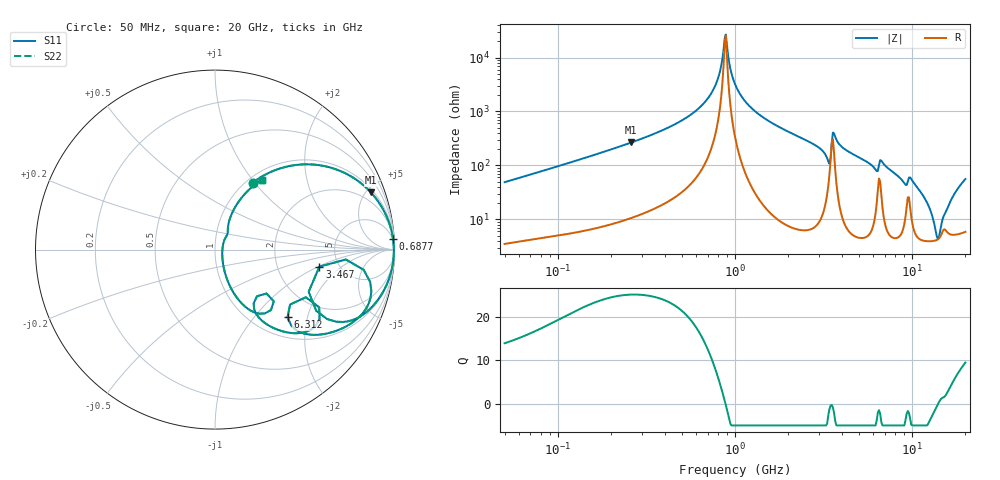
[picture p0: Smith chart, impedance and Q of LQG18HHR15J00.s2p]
!Murata Part Number: LQG18HHR15J00
!These Parameters are Measured in Series Mode Connection
!  o--[Z]--o
!Port1  Port2
!  o-------o
!Freq. Start=50[MHz] Stop=20[GHz], 401[Steps]
# Hz S RI R 50
!Freq.(Hz) S11(Real) S11(Imag) S21(Real) S21(Imag) S12(Real) S12(Imag) S22(Real) S22(Imag)
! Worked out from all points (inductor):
!   401 points, 50 MHz to 20 GHz, reference 50 ohm
!   read as one part in series: L = 153 nH near 51.52 MHz
!   highest Q = 25.1 at 259.7 MHz (marker M1), where L = 163 nH
!   self-resonance near 873.9 MHz
!   S11 on the Smith chart (normalised r, x): 50 MHz: 1.07, +0.98; 687.7 MHz: 3, +32; 3.467 GHz: 3.55, -1.03; 6.312 GHz: 1.40, -1.52; 20 GHz: 1.12, +1.12
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5e7  0.2095 0.3726  0.7905 -0.3726  0.7905 -0.3726  0.2095 0.3726
1.364002e8  0.631 0.4603  0.369 -0.4603  0.369 -0.4603  0.631 0.4603
2.597386e8  0.8669 0.3203  0.1331 -0.3203  0.1331 -0.3203  0.8669 0.3203
3.721004e8  0.9385 0.2206  0.0615 -0.2206  0.0615 -0.2206  0.9385 0.2206
6.87656e8  0.9915 0.0615  0.00849 -0.0615  0.00849 -0.0615  0.9915 0.0615
7.868965e8  0.9952 0.0284  0.00484 -0.0284  0.00484 -0.0284  0.9952 0.0284
8.870719e8  0.9964 -0.000985  0.00359 0.000985  0.00359 0.000985  0.9964 -0.000985
1e9  0.9958 -0.0306  0.00421 0.0306  0.00421 0.0306  0.9958 -0.0306
1.369645e9  0.9843 -0.1118  0.0157 0.1118  0.0157 0.1118  0.9843 -0.1118
2.728004e9  0.861 -0.3331  0.139 0.3331  0.139 0.3331  0.861 -0.3331
3.216634e9  0.7123 -0.4034  0.2877 0.4034  0.2877 0.4034  0.7123 -0.4034
3.466789e9  0.5817 -0.0949  0.4183 0.0949  0.4183 0.0949  0.5817 -0.0949
3.736399e9  0.8662 -0.27  0.1338 0.27  0.1338 0.27  0.8662 -0.27
5.194772e9  0.6327 -0.4654  0.3673 0.4654  0.3673 0.4654  0.6327 -0.4654
6.311513e9  0.404 -0.3774  0.596 0.3774  0.596 0.3774  0.404 -0.3774
6.802353e9  0.5577 -0.4282  0.4423 0.4282  0.4423 0.4282  0.5577 -0.4282
7.442007e9  0.4228 -0.4644  0.5772 0.4644  0.5772 0.4644  0.4228 -0.4644
1.098561e10  0.1359 -0.2853  0.8641 0.2853  0.8641 0.2853  0.1359 -0.2853
1.238412e10  0.0641 -0.1569  0.9359 0.1569  0.9359 0.1569  0.0641 -0.1569
1.396067e10  0.0408 -0.00708  0.9592 0.00708  0.9592 0.00708  0.0408 -0.00708
1.670968e10  0.0938 0.2004  0.9062 -0.2004  0.9062 -0.2004  0.0938 0.2004
2e10  0.2608 0.3895  0.7392 -0.3895  0.7392 -0.3895  0.2608 0.3895
